| Philips Semiconductors Inc.
| Logic Products Group
| IBIS model of 74LVC244A
|  OCTAL BUFFER/LINE DRIVER; 3-STATE; 5-VOLT TOLERANT
|[Packages]:
|[Package1]: SO 20-pin (D) Package ;
|[Package2]: SSOP 20-Pin Packages ;
|[Package3]: TSSOP 20-pin (PW) Package ;
|[Package4]: DQFN 20-Pin Package ;
[IBIS Ver]   3.2
[File Name]   lvc244a.ibs
[File Rev]   1.2
[Date]   26-Nov-2002
[Source]   File created from simulations by LPG
   Philips Semiconductors Nijmegen
[Notes]   V1.2   Ibis model.
| Remark:
| The Power Clamp curves have been omitted since there is no power clamp diode.
| Revision History
| Version Date   Author/ Description
|   Editor
| 1.0   1999   Initial Version
| 1.1   November 2001 RM   Revised for Ibis 3.2:
|   Added Model Spec and Model Selector
| 1.2   November 2002 RM   Revised: Power Clamp curves omitted, constant
|   end points for Ground Clamp and V/t curves.
|   Added DQFN package.
[Disclaimer]
   (C) Copyright 2002 Philips Semiconductors
   All rights reserved
   Philips Semiconductors warrants and represents that the IBIS model
   identified herein is owned by Philips Semiconductors (PHILIPS). The
   model provided is not warranted as fully representing all of the
   operating characteristics and specifications of the semiconductor
   products to which the model relates.  Moreover, unless there is a
   signed, written agreement to the contrary, this IBIS model is
   furnished on an "as is" basis without support or warranty of any
   kind, either expressed or implied, regarding the use thereof, and
   PHILIPS specifically disclaims all implied warranties of
   merchantability and fitness of the model for any purpose.
   PHILIPS does not assume any liability arising out of the application
   or use of this IBIS model including infringement of patents and
   copyrights, nor does PHILIPS convey any license under its patents and
   copyrights or the rights of others.
   PHILIPS provides IBIS models as a service to our customers. You and
   your company shall not distribute, convey, sell, or give these models
   to anyone else without receiving prior written permission from
   PHILIPS.
   PHILIPS reserves the right to make changes without notice to these
   IBIS models to improve reliability, function, or design.
   Please be aware that your receipt and subsequent use of the IBIS
   information provided shall serve as acceptance of the terms and
   conditions of this agreement.  If you do not accept these terms,
   you should return or destroy the IBIS models and any other
   accompanying information immediately.
| to specify a consistent format that can be parsed by software, allowing
| simulation vendors to derive models compatible with their own products.
| One goal of this template is to represent the current state of IBIS data,
| while allowing a growth path to more complex models / methods (when deemed
| appropriate).  This would be accomplished by a revision of the base
| template, and possibly the addition of new keywords or categories.
| Another goal of this template is to ensure that it is simple enough for
| semiconductor vendors and customers to use and modify, while ensuring that
| it is rigid enough for simulation vendors to write reliable parsers.
| Finally, this template is meant to contain a complete description of the I/O
| elements on an entire component.  Consequently, several models will need to
| be defined in each file, as well as a table that equates the appropriate
| buffer to the correct pin and signal name.
| Version 3.2 of this electronic template was finalized by an industry-wide
| group of experts representing various companies and interests.  Regular
| "EIA IBIS Open Forum" meetings were held to accomplish this task.
| Commitment to Backward Compatibility.  Version 1.0 is the first valid IBIS
| ASCII file format.  It represents the minimum amount of I/O buffer
| information required to create an accurate IBIS model of common CMOS and
| bipolar I/O structures.  Future revisions of the ASCII file will add items
| considered to be "enhancements" to Version 1.0 to allow accurate modeling
| of new, or other I/O buffer structures.  Consequently, all future revisions
| will be considered supersets of Version 1.0, allowing backward
| compatibility.  In addition, as modeling platforms develop support for
| revisions of the IBIS ASCII template, all previous revisions of the template
| must also be supported.
| Version 1.1 update.  The file "ver1_1.ibs" is conceptually the same as the
| 1.0 version of the IBIS ASCII format (ver1_0.ibs).  However, various
| comments have been added for further clarification.
| Version 2.0 update.  The file "ver2_0.ibs" maintains backward compatibility
| with Versions 1.0 and 1.1.  All new keywords and elements added in Version
| 2.0 are optional.  A complete list of changes to the specification is in the
| IBIS Version 2.0 Release Notes document ("ver2_0.rn").
| Version 2.1 update.  The file "ver2_1.ibs" contains clarification text
| changes, corrections, and two additional waveform parameters beyond
| Version 2.0.
| Version 3.0 update.  The file "ver3_0.ibs" adds a number of new keywords
| and functionality.  A complete list of functions can be found on eda.org
| under /pub/ibis/birds/birddir.txt showing the approved Buffer Issue
| Resolution Documents (BIRDs) that have been approved for Version 3.0.
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[Component]   74LVC244A_1
[Manufacturer]   Philips Semiconductors Inc.
[Package]
|   typ   min   max
R_pkg   5.95E-02   5.36E-02   6.59E-02
L_pkg   4.21E-09   3.07E-09   5.91E-09
C_pkg   0.910E-12  0.758E-12  1.110E-12
[Pin] signal_name   model_name   R_pin   L_pin   C_pin
   1   1OE#   lvc_in2 5.75E-02 5.91E-09 1.050E-12
   2   1A0   lvc_in2 6.25E-02 4.85E-09 1.040E-12
   3   2Y0   lvc_tristn 6.59E-02 3.92E-09 0.861E-12
   4   1A1   lvc_in2 5.79E-02 3.32E-09 0.803E-12
   5   2Y1   lvc_tristn 5.36E-02 3.07E-09 0.758E-12
   6   1A2   lvc_in2 5.36E-02 3.07E-09 0.758E-12
   7   2Y2   lvc_tristn 5.79E-02 3.32E-09 0.803E-12
   8   1A3   lvc_in2 6.59E-02 3.92E-09 0.861E-12
   9   2Y3   lvc_tristn 6.25E-02 4.85E-09 1.040E-12
   10   GND   GND 5.75E-02 5.91E-09 1.110E-12
   11   2A3   lvc_in2 5.75E-02 5.91E-09 1.110E-12
   12   1Y3   lvc_tristn 6.25E-02 4.85E-09 1.040E-12
   13   2A2   lvc_in2 6.59E-02 3.92E-09 0.861E-12
   14   1Y2   lvc_tristn 5.79E-02 3.32E-09 0.803E-12
   15   2A1   lvc_in2 5.36E-02 3.07E-09 0.758E-12
   16   1Y1   lvc_tristn 5.36E-02 3.07E-09 0.758E-12
   17   2A0   lvc_in2 5.79E-02 3.32E-09 0.803E-12
   18   1Y0   lvc_tristn 6.59E-02 3.92E-09 0.861E-12
   19   2OE#   lvc_in2 6.25E-02 4.85E-09 1.040E-12
   20   VCC   POWER 5.75E-02 5.91E-09 1.110E-12
|   Info for  SSOP 20-Pin Packages
[Component]   74LVC244A_2
[Manufacturer]   Philips Semiconductors Inc.
[Package]
|   typ   min   max
R_pkg   50.90E-03   43.00E-03   62.10E-03
L_pkg   2.37E-09   1.87E-09   3.04E-09
C_pkg   0.62E-12   0.55E-12   0.71E-12
[Pin] signal_name   model_name   R_pin   L_pin   C_pin
   1   1OE#   lvc_in2 47.20E-03 3.04E-09 0.65E-12
   2   1A0   lvc_in2 51.40E-03 2.60E-09 0.70E-12
   3   2Y0   lvc_tristn 62.10E-03 2.31E-09 0.59E-12
   4   1A1   lvc_in2 50.80E-03 2.03E-09 0.58E-12
   5   2Y1   lvc_tristn 43.00E-03 1.87E-09 0.56E-12
   6   1A2   lvc_in2 43.00E-03 1.87E-09 0.56E-12
   7   2Y2   lvc_tristn 50.80E-03 2.03E-09 0.58E-12
   8   1A3   lvc_in2 62.10E-03 2.31E-09 0.59E-12
   9   2Y3   lvc_tristn 51.40E-03 2.60E-09 0.70E-12
   10   GND   GND 47.20E-03 3.04E-09 0.69E-12
   11   2A3   lvc_in2 47.20E-03 3.05E-09 0.69E-12
   12   1Y3   lvc_tristn 51.40E-03 2.60E-09 0.70E-12
   13   2A2   lvc_in2 62.10E-03 2.32E-09 0.59E-12
   14   1Y2   lvc_tristn 50.80E-03 2.03E-09 0.58E-12
   15   2A1   lvc_in2 43.00E-03 1.88E-09 0.55E-12
   16   1Y1   lvc_tristn 43.00E-03 1.87E-09 0.55E-12
   17   2A0   lvc_in2 50.80E-03 2.03E-09 0.58E-12
   18   1Y0   lvc_tristn 62.10E-03 2.31E-09 0.59E-12
   19   2OE#   lvc_in2 51.40E-03 2.60E-09 0.71E-12
   20   VCC   POWER 47.50E-03 3.00E-09 0.68E-12
|   Info for  TSSOP 20-pin (PW) Package
[Component]   74LVC244A_3
[Manufacturer]   Philips Semiconductors Inc.
[Package]
|   typ   min   max
R_pkg   7.24E-02   6.63E-02   8.34E-02
L_pkg   2.47E-09   2.09E-09   3.18E-09
C_pkg   0.341E-12  0.282E-12  0.420E-12
[Pin] signal_name   model_name   R_pin   L_pin   C_pin
   1   1OE#   lvc_in2 6.63E-02 3.18E-09 0.408E-12
   2   1A0   lvc_in2 6.67E-02 2.55E-09 0.398E-12
   3   2Y0   lvc_tristn 8.34E-02 2.35E-09 0.317E-12
   4   1A1   lvc_in2 7.44E-02 2.16E-09 0.293E-12
   5   2Y1   lvc_tristn 7.10E-02 2.09E-09 0.282E-12
   6   1A2   lvc_in2 7.10E-02 2.09E-09 0.282E-12
   7   2Y2   lvc_tristn 7.44E-02 2.16E-09 0.293E-12
   8   1A3   lvc_in2 8.34E-02 2.35E-09 0.317E-12
   9   2Y3   lvc_tristn 6.67E-02 2.55E-09 0.397E-12
   10   GND   GND 6.63E-02 3.18E-09 0.420E-12
   11   2A3   lvc_in2 6.63E-02 3.17E-09 0.420E-12
   12   1Y3   lvc_tristn 6.67E-02 2.55E-09 0.397E-12
   13   2A2   lvc_in2 8.34E-02 2.35E-09 0.317E-12
   14   1Y2   lvc_tristn 7.44E-02 2.16E-09 0.293E-12
   15   2A1   lvc_in2 7.10E-02 2.09E-09 0.282E-12
   16   1Y1   lvc_tristn 7.10E-02 2.09E-09 0.282E-12
   17   2A0   lvc_in2 7.44E-02 2.16E-09 0.293E-12
   18   1Y0   lvc_tristn 8.34E-02 2.35E-09 0.317E-12
   19   2OE#   lvc_in2 6.67E-02 2.55E-09 0.398E-12
   20   VCC   POWER 6.63E-02 3.17E-09 0.420E-12
|   Info for  DQFN 20-Pin Package
[Component]   74LVC244A_4
[Manufacturer]   Philips Semiconductors Inc.
[Package]
|   typ   min   max
R_pkg   9.3470E-02   5.7002E-02   1.2474E-01
L_pkg   1.056E-09   6.200E-10   1.430E-09
C_pkg   6.45E-14   4.70E-14   8.70E-14
[Pin] signal_name   model_name   R_pin   L_pin   C_pin
   1   1OE#   lvc_in2 1.25E-01 1.40E-09 8.10E-14
   2   1A0   lvc_in2 9.39E-02 1.06E-09 5.60E-14
   3   2Y0   lvc_tristn 6.75E-02 7.73E-10 5.00E-14
   4   1A1   lvc_in2 5.84E-02 6.20E-10 4.80E-14
   5   2Y1   lvc_tristn 5.92E-02 6.31E-10 4.90E-14
   6   1A2   lvc_in2 6.86E-02 7.74E-10 5.10E-14
   7   2Y2   lvc_tristn 9.66E-02 1.07E-09 5.70E-14
   8   1A3   lvc_in2 1.24E-01 1.40E-09 7.90E-14
   9   2Y3   lvc_tristn 1.24E-01 1.41E-09 8.70E-14
   10   GND   GND 1.24E-01 1.43E-09 8.70E-14
   11   2A3   lvc_in2 1.24E-01 1.41E-09 8.10E-14
   12   1Y3   lvc_tristn 9.07E-02 1.05E-09 5.60E-14
   13   2A2   lvc_in2 6.94E-02 7.85E-10 5.00E-14
   14   1Y2   lvc_tristn 5.70E-02 6.28E-10 4.70E-14
   15   2A1   lvc_in2 5.87E-02 6.28E-10 4.90E-14
   16   1Y1   lvc_tristn 7.06E-02 8.02E-10 5.10E-14
   17   2A0   lvc_in2 9.24E-02 1.07E-09 5.70E-14
   18   1Y0   lvc_tristn 1.21E-01 1.39E-09 8.10E-14
   19   2OE#   lvc_in2 1.22E-01 1.39E-09 8.70E-14
   20   VCC   POWER 1.23E-01 1.41E-09 8.50E-14
[Model Selector]   lvc_in2
| Remark: If your software does not support the Model Selector
|   Please comment out the lines of the Model Selector, which
|   contain the name of the Model, except the one you want to use.
LVC_IN2_33   3.3V-Vcc input model
LVC_IN2_25   2.5V-Vcc input model
[Model Selector]   lvc_tristn
| Remark: If your software does not support the Model Selector
|   Please comment out the lines of the Model Selector, which
|   contain the name of the Model, except the one you want to use.
LVC_TRISTN_33   3.3V-Vcc tristate output model, non-inverting
LVC_TRISTN_25   2.5V-Vcc tristate output model, non-inverting
| Models and submodels in the file (4): LVC_IN2_33 (Input), LVC_IN2_25 (Input), LVC_TRISTN_33 (3-state), LVC_TRISTN_25 (3-state)
